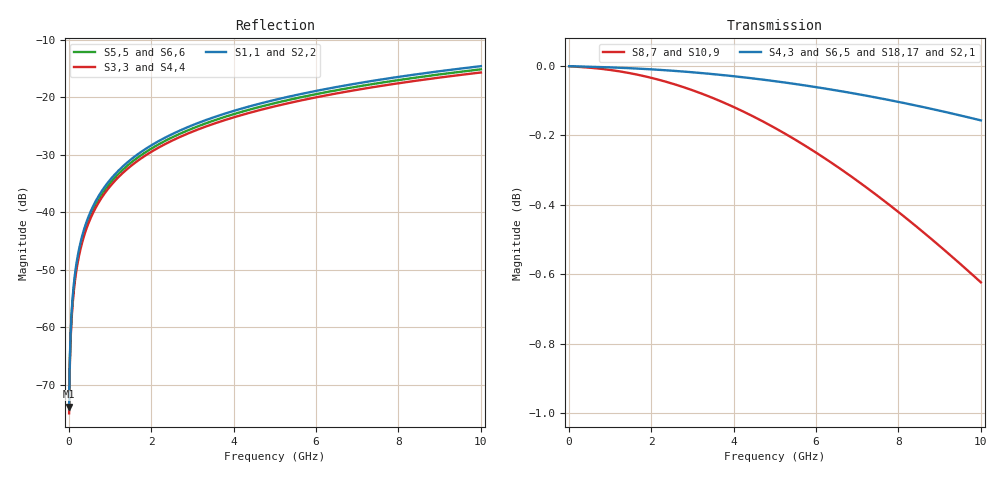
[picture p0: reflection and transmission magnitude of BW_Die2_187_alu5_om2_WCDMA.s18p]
! Created Fri Sep 09 10:46:31 2011
! 18 Port Network Data from SP1.SP block
! freq  magS1_1  angS1_1  magS1_2  angS1_2  magS1_3  angS1_3  magS1_4  angS1_4
!  magS1_5  angS1_5  magS1_6  angS1_6  magS1_7  angS1_7  magS1_8  angS1_8
!  magS1_9  angS1_9  magS1_10  angS1_10  magS1_11  angS1_11  magS1_12  angS1_12
!  magS1_13  angS1_13  magS1_14  angS1_14  magS1_15  angS1_15  magS1_16  angS1_16
!  magS1_17  angS1_17  magS1_18  angS1_18
!  magS2_1  angS2_1  magS2_2  angS2_2
!  magS2_3  angS2_3  magS2_4  angS2_4  magS2_5  angS2_5  magS2_6  angS2_6
!  magS2_7  angS2_7  magS2_8  angS2_8  magS2_9  angS2_9  magS2_10  angS2_10
!  magS2_11  angS2_11  magS2_12  angS2_12  magS2_13  angS2_13  magS2_14  angS2_14
!  magS2_15  angS2_15  magS2_16  angS2_16  magS2_17  angS2_17  magS2_18  angS2_18
!  magS3_1  angS3_1  magS3_2  angS3_2  magS3_3  angS3_3  magS3_4  angS3_4
!  magS3_5  angS3_5  magS3_6  angS3_6  magS3_7  angS3_7  magS3_8  angS3_8
!  magS3_9  angS3_9  magS3_10  angS3_10  magS3_11  angS3_11  magS3_12  angS3_12
!  magS3_13  angS3_13  magS3_14  angS3_14  magS3_15  angS3_15  magS3_16  angS3_16
!  magS3_17  angS3_17  magS3_18  angS3_18
!  magS4_1  angS4_1  magS4_2  angS4_2
!  magS4_3  angS4_3  magS4_4  angS4_4  magS4_5  angS4_5  magS4_6  angS4_6
!  magS4_7  angS4_7  magS4_8  angS4_8  magS4_9  angS4_9  magS4_10  angS4_10
!  magS4_11  angS4_11  magS4_12  angS4_12  magS4_13  angS4_13  magS4_14  angS4_14
!  magS4_15  angS4_15  magS4_16  angS4_16  magS4_17  angS4_17  magS4_18  angS4_18
!  magS5_1  angS5_1  magS5_2  angS5_2  magS5_3  angS5_3  magS5_4  angS5_4
!  magS5_5  angS5_5  magS5_6  angS5_6  magS5_7  angS5_7  magS5_8  angS5_8
!  magS5_9  angS5_9  magS5_10  angS5_10  magS5_11  angS5_11  magS5_12  angS5_12
!  magS5_13  angS5_13  magS5_14  angS5_14  magS5_15  angS5_15  magS5_16  angS5_16
!  magS5_17  angS5_17  magS5_18  angS5_18
!  magS6_1  angS6_1  magS6_2  angS6_2
!  magS6_3  angS6_3  magS6_4  angS6_4  magS6_5  angS6_5  magS6_6  angS6_6
!  magS6_7  angS6_7  magS6_8  angS6_8  magS6_9  angS6_9  magS6_10  angS6_10
!  magS6_11  angS6_11  magS6_12  angS6_12  magS6_13  angS6_13  magS6_14  angS6_14
!  magS6_15  angS6_15  magS6_16  angS6_16  magS6_17  angS6_17  magS6_18  angS6_18
!  magS7_1  angS7_1  magS7_2  angS7_2  magS7_3  angS7_3  magS7_4  angS7_4
!  magS7_5  angS7_5  magS7_6  angS7_6  magS7_7  angS7_7  magS7_8  angS7_8
!  magS7_9  angS7_9  magS7_10  angS7_10  magS7_11  angS7_11  magS7_12  angS7_12
!  magS7_13  angS7_13  magS7_14  angS7_14  magS7_15  angS7_15  magS7_16  angS7_16
!  magS7_17  angS7_17  magS7_18  angS7_18
!  magS8_1  angS8_1  magS8_2  angS8_2
!  magS8_3  angS8_3  magS8_4  angS8_4  magS8_5  angS8_5  magS8_6  angS8_6
!  magS8_7  angS8_7  magS8_8  angS8_8  magS8_9  angS8_9  magS8_10  angS8_10
!  magS8_11  angS8_11  magS8_12  angS8_12  magS8_13  angS8_13  magS8_14  angS8_14
!  magS8_15  angS8_15  magS8_16  angS8_16  magS8_17  angS8_17  magS8_18  angS8_18
!  magS9_1  angS9_1  magS9_2  angS9_2  magS9_3  angS9_3  magS9_4  angS9_4
!  magS9_5  angS9_5  magS9_6  angS9_6  magS9_7  angS9_7  magS9_8  angS9_8
!  magS9_9  angS9_9  magS9_10  angS9_10  magS9_11  angS9_11  magS9_12  angS9_12
!  magS9_13  angS9_13  magS9_14  angS9_14  magS9_15  angS9_15  magS9_16  angS9_16
!  magS9_17  angS9_17  magS9_18  angS9_18
!  magS10_1  angS10_1  magS10_2  angS10_2
!  magS10_3  angS10_3  magS10_4  angS10_4  magS10_5  angS10_5  magS10_6  angS10_6
!  magS10_7  angS10_7  magS10_8  angS10_8  magS10_9  angS10_9  magS10_10  angS10_10
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# ghz S ma R 50
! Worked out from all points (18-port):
!   1000 points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, 10 MHz to 10 GHz, reference 50 ohm
!   strongest paths, dB at 10 MHz, 2.51 GHz, 5.01 GHz, 7.51 GHz, 10 GHz:
!     S4,3: 0.0, 0.0, 0.0, -0.1, -0.2
!     S6,5: 0.0, 0.0, 0.0, -0.1, -0.2
!     S18,17: 0.0, 0.0, 0.0, -0.1, -0.2
!     S2,1: 0.0, 0.0, -0.1, -0.1, -0.2
!     S8,7: 0.0, -0.1, -0.2, -0.4, -0.6
!     S10,9: 0.0, -0.1, -0.2, -0.4, -0.6
!   lowest |S11| = -73.8 dB at 10 MHz (marker M1), VSWR 1.00, Z = 50 + j0.0191 ohm
!   |S11| at or under -10 dB: start of sweep to end of sweep
